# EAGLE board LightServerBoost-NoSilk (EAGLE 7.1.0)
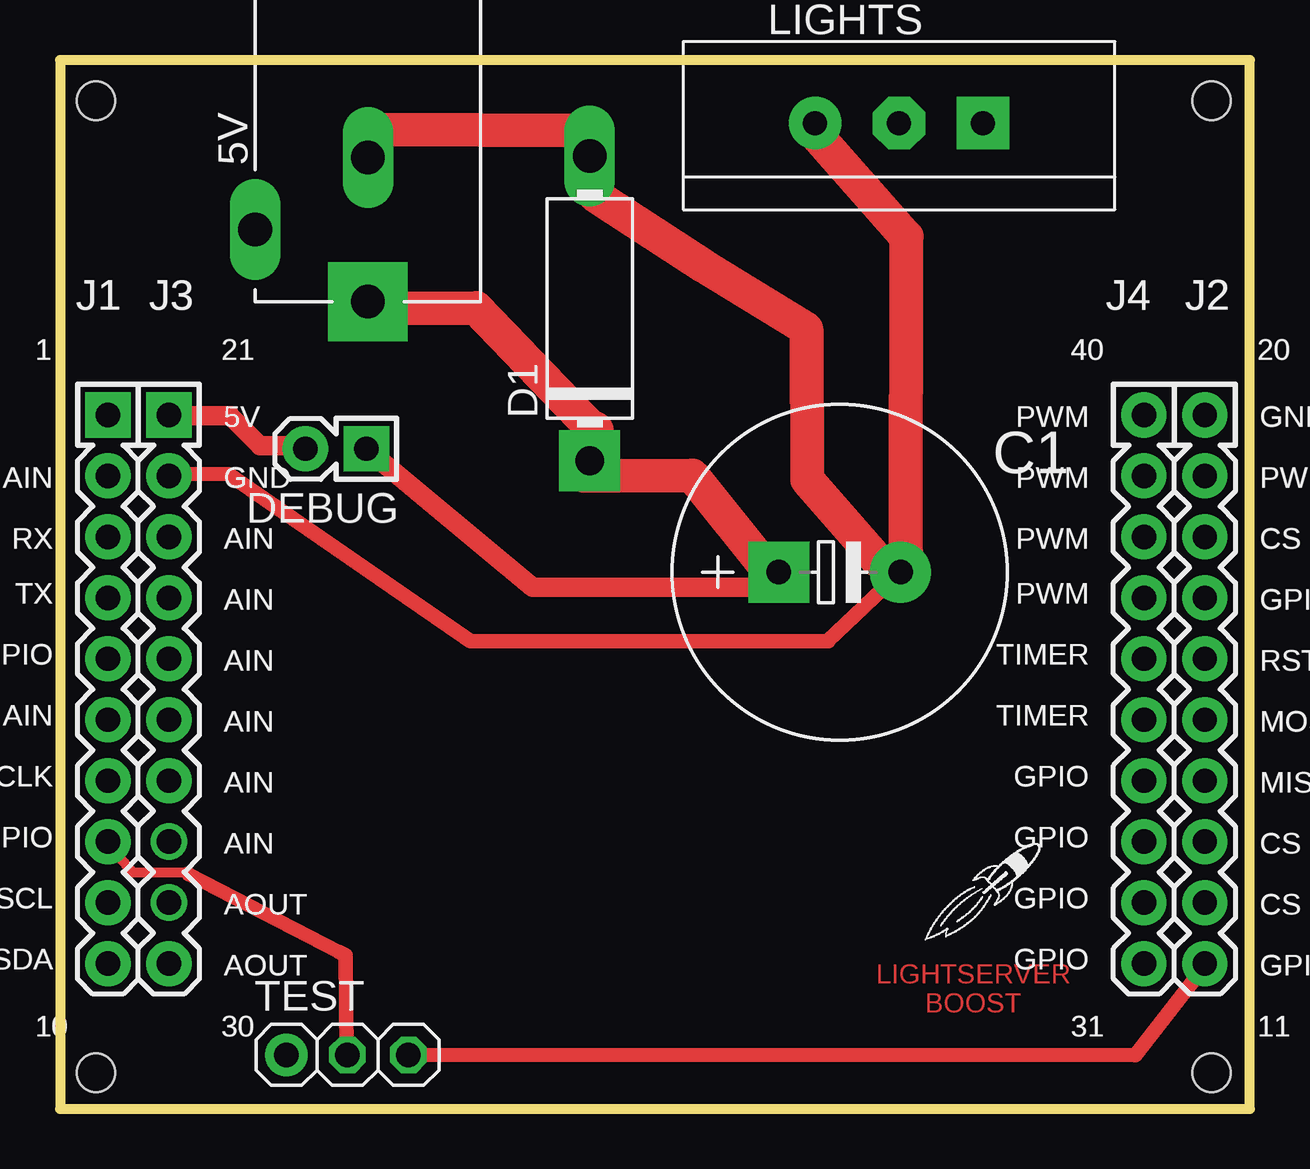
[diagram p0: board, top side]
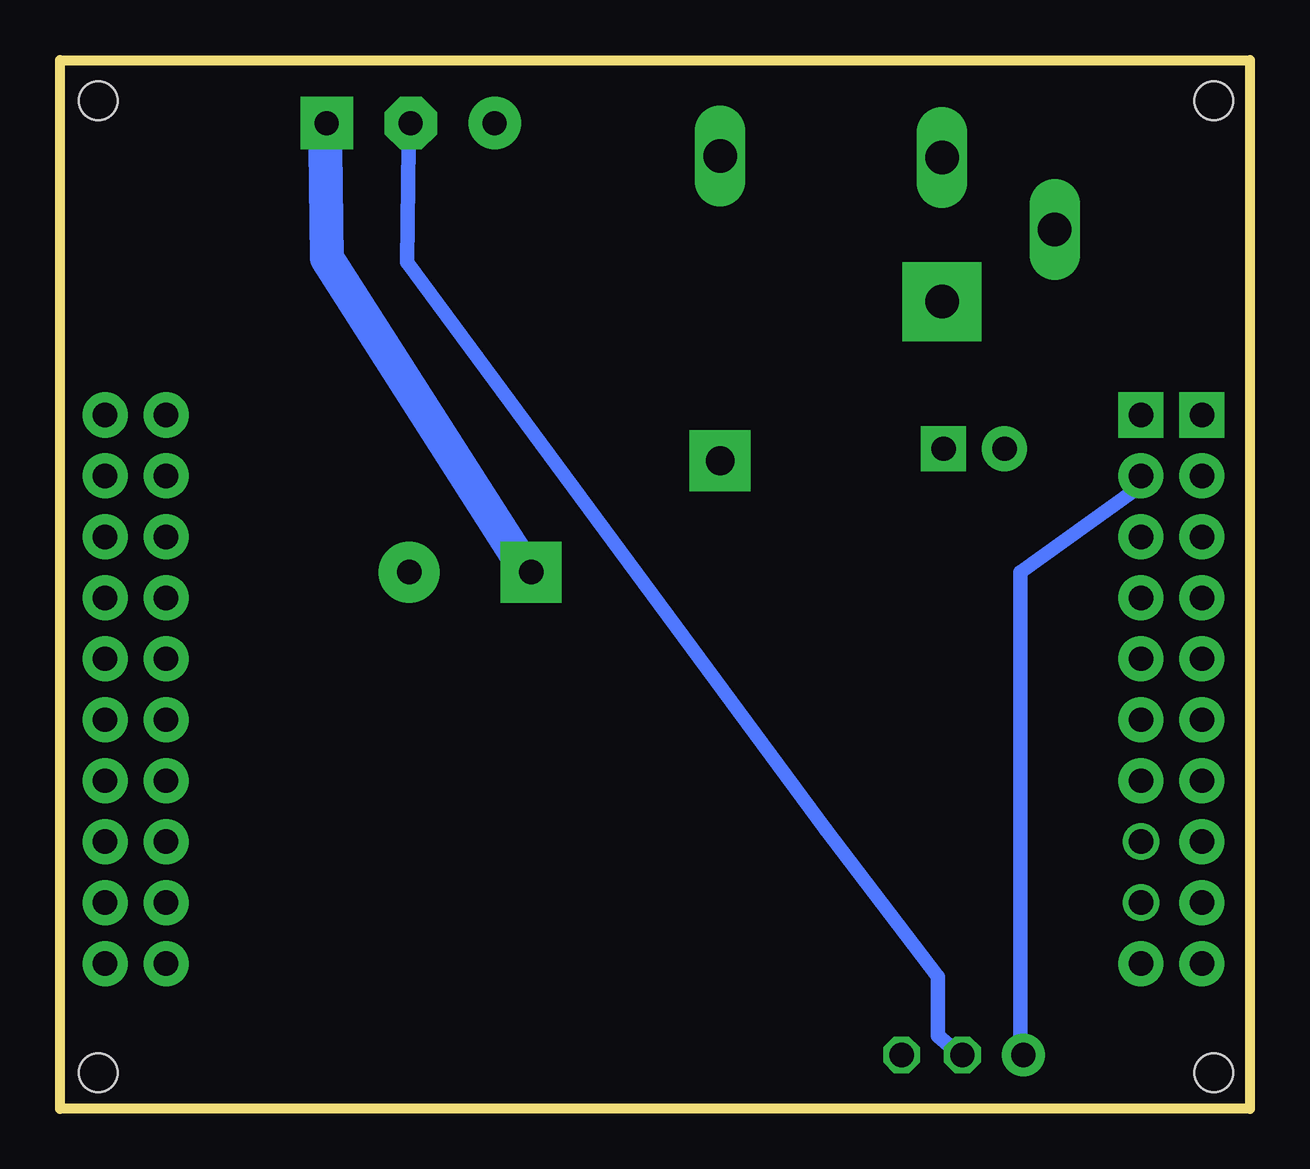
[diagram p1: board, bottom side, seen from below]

Size 49.6 x 43.7 mm. Coordinates in mm from the lower left corner, seen from the top.
Outline: 0,0 49.6,0 49.6,43.7 0,43.7 0,0
Copper layers (1*16): Top 0.035mm / dielectric 1.5mm / Bottom 0.035mm
Design rules "SeeedStudio_2layer_DRU_no_angle_20140221": minimum track width 6mil, minimum drill 12mil, track to track 6mil, track to pad 6mil, pad to pad 6mil, via to via 6mil, smd to smd 0mil, copper to edge 10mil, drill to drill 10mil, minimum pad ring 10mil, minimum via ring 6mil, stop-mask expansion 2mil, vias tented up to drill 100mil, thermal gap 10mil
Holes 1.6 mm at 1.5,1.5 1.5,42 48,1.5 48,42

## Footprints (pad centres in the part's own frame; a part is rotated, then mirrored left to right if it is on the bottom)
PJ-102AH = drill 1.4 pad 3.302 square: 1 0,-3 | drill 1.4 long: 2 0,3; 3 -4.7,0
E5-13 = drill 1.016 pad 2.54 square: + -2.54,0 | drill 1.016 pad 2.54: - 2.54,0
CB417-12 = drill 1.397 long: A 6.35,0 | drill 1.2 pad 2.54 square: C -6.35,0
1X02 = drill 1.016 pad 1.88 square: 1 -1.27,0 | drill 1.016 pad 1.88: 2 1.27,0
4X10-BOOSTERPACK = drill 1.016 pad 1.88 square: 1 0,10.16; 21 2.54,10.16 | drill 1.016 pad 1.88: 2 0,7.62; 3 0,5.08; 4 0,2.54; 5 0,0; 6 0,-2.54; 7 0,-5.08; 8 0,-7.62; 9 0,-10.16; 10 0,-12.7; 11 45.72,-12.7; 12 45.72,-10.16; 13 45.72,-7.62; 14 45.72,-5.08; 15 45.72,-2.54; 16 45.72,0; 17 45.72,2.54; 18 45.72,5.08; 19 45.72,7.62; 20 45.72,10.16; 22 2.54,7.62; 23 2.54,5.08; 24 2.54,2.54; 25 2.54,0; 26 2.54,-2.54; 27 2.54,-5.08; 30 2.54,-12.7; 31 43.18,-12.7; 32 43.18,-10.16; 33 43.18,-7.62; 34 43.18,-5.08; 35 43.18,-2.54; 36 43.18,0; 37 43.18,2.54; 38 43.18,5.08; 39 43.18,7.62; 40 43.18,10.16 | drill 1.016 pad 1.422: 28 2.54,-7.62; 29 2.54,-10.16
1X3-3.5MM = drill 1 pad 2.184 square: 1 3.5,0 | drill 1 pad 2.184 octagon: 2 0,0 | drill 1 pad 2.184: 3 -3.5,0
1X03 = drill 1.016 pad 1.778: 1 -2.54,0 | drill 1.016 octagon: 2 0,0; 3 2.54,0

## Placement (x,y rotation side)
5V  [PJ-102AH]  12.84,36.63 0 top
C1  [E5-13]  32.5,22.36 0 top
D1  [CB417-12]  22.08,33.35 90 top
DEBUG  [1X02]  11.5,27.5 180 top  (not fitted)
E$1  [4X10-BOOSTERPACK]  2,18.75 0 top  (not fitted)
E$2  [LOGO-ROCKET]  38.61,9.23 0 top
E$5  [4X10-BOOSTERPACK]  2,18.75 0 top  (not fitted)
LIGHTS  [1X3-3.5MM]  34.98,41.07 0 top
TEST  [1X03]  11.98,2.25 0 top

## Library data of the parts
5V = connectors
C1 LIGHTS TEST = adafruit
D1 = ref-packages
DEBUG E$1 E$2 E$5 = EAGLE_BoosterPack_Library

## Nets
S$2: C1.-

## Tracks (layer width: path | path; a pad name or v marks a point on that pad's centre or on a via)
LIGHTSERVERBOOST
  Bottom 0.61: 12.11,2.28 13,3.03 13,5.5 17.68,11.62 35.13,35.28 35.08,40.14
S$1
  Bottom 1.422: 30.16,22.44 38.47,35.44 38.53,40
S$2
  Top 0.61: C1.- 32,19.5 32.04,19.48 17.11,19.48 7.03,26.44 4.46,26.45
S$3
  Top 0.406: 3,9.86 5.25,9.86
S$4
  Top 1.422: 22.25,28.25 17.35,33.36 13.03,33.34
  Top 1.676: 22.25,28.21 22.25,28.25
S$5
  Top 0.406: 2,11 3,9.9
S$6
  Bottom 0.61: 4.79,25.79 9.57,22.36 9.57,2.22
S$7
  Top 0.813: 12.75,27.5 19.7,21.72 28.83,21.73
S$8
  Top 0.61: 14.5,2.25 44.81,2.23 47.75,6
S$9
  Top 0.813: 4.76,28.87 7.1,28.87 8.35,27.62 10.01,27.62
S$10
  Top 1.422: 12.73,40.81 22.35,40.77
S$11
  Top 1.422: 21.81,26.38 26.35,26.39 29.53,22.42
S$12
  Top 0.406: 22,38.5 22.29,38.08
  Top 1.422: 22.29,38.08 26.83,35.12 31.11,32.5 31.14,26.22 34.07,22.86
S$13
  Top 1.422: 31.56,40.57 35.28,36.34 35.27,23.19
S$14
  Top 0.61: 5.37,9.77 11.6,6.55 11.91,6.39 11.96,2.32

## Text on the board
Top: LIGHTSERVER / BOOST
